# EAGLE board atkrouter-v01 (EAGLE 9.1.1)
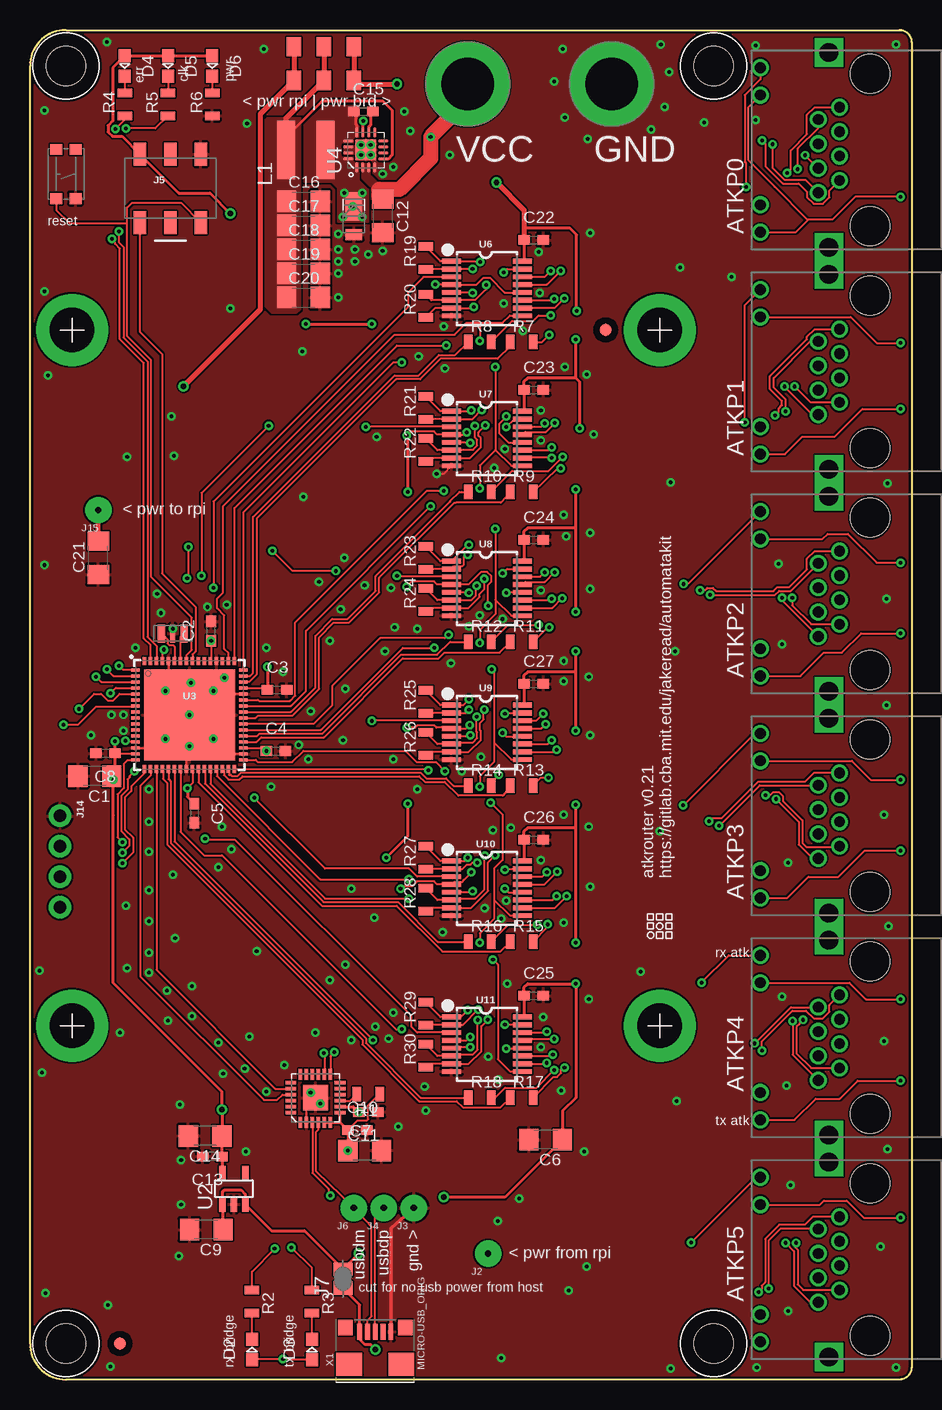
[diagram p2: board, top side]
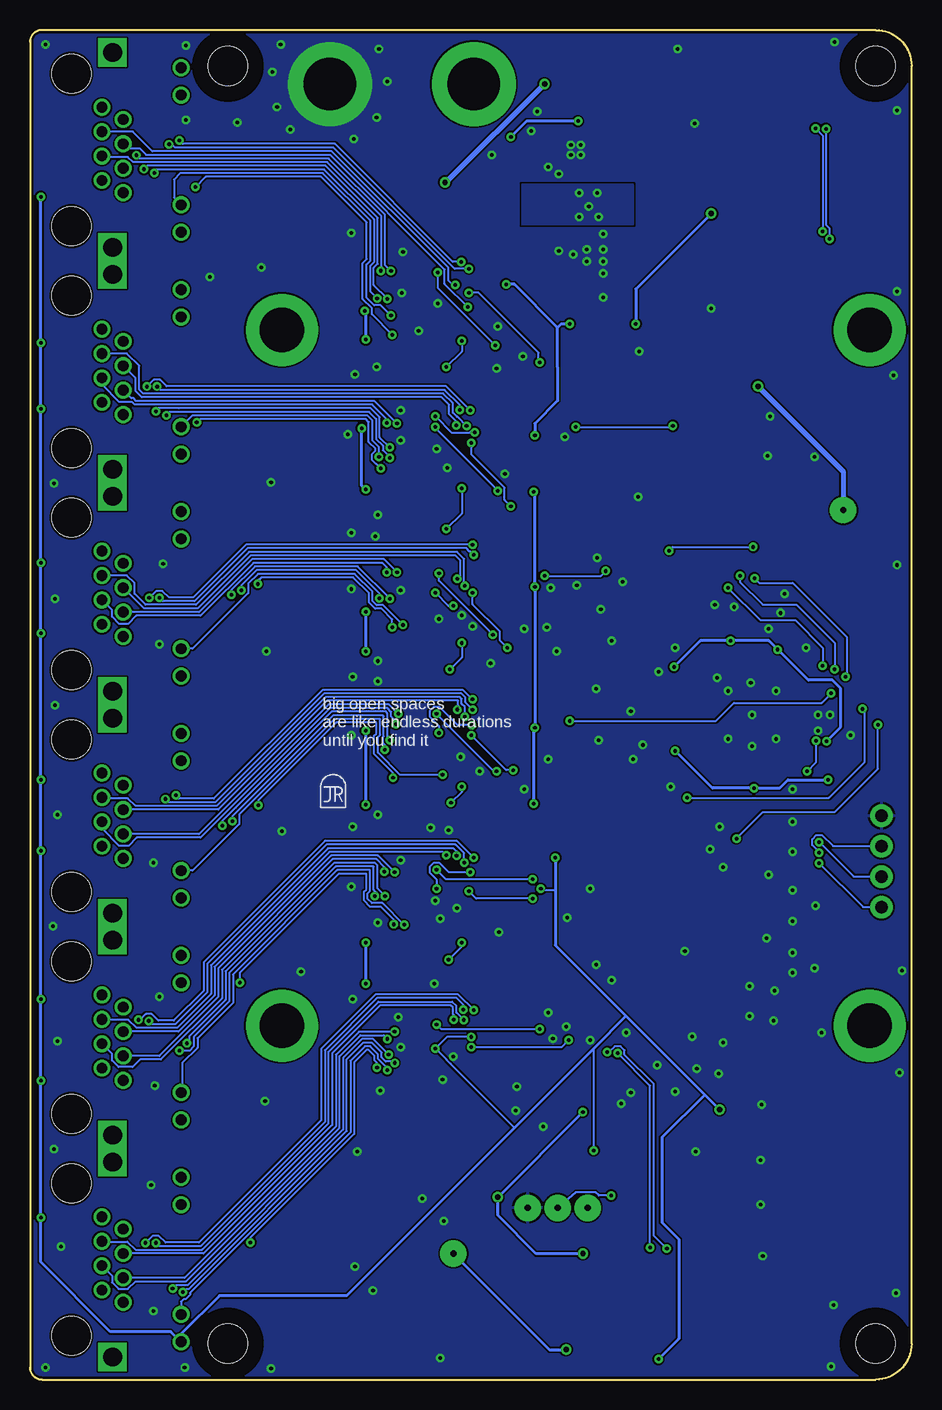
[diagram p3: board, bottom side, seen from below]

Size 73.5 x 112.5 mm. Coordinates in mm from the lower left corner, seen from the top.
Outline: 72.5,0 3,0 arc-90 0,3 0,109.5 arc-90 3,112.5 72.5,112.5 arc-90 73.5,111.5 73.5,1 arc-90 72.5,0
Copper layers (1*16): Top 0.035mm / dielectric 1.5mm / Bottom 0.035mm
Design rules "default *": minimum track width 6mil, minimum drill 0.3mm, track to track 6mil, track to pad 6mil, pad to pad 6mil, via to via 6mil, smd to smd 6mil, copper to edge 8mil, drill to drill 6mil, minimum pad ring 10mil, minimum via ring 8mil, stop-mask expansion 4mil, vias tented up to drill 25mil, thermal gap 8mil

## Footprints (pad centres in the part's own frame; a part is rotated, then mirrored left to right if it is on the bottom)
1206 = smd 1.6 x 1.8: 1 -1.4,0; 2 1.4,0
0603-CAP = smd 0.96 x 0.8: 1 -0.8,0; 2 0.8,0
SOD-123HE = smd 2.4 x 1.4: P$1 0.8,0 | smd 0.9 x 1.4: P$2 -1.55,0
LED0805 = smd 1.1 x 1: 1 -0.85,0; 2 0.85,0
FIDUCIAL_1MM = smd 1 x 1: 1 0,0
POGO = drill 0.51 pad 2.184: P$1 0,0
PDI_2X3_SMD = smd 1.02 x 1.9: 1 -2.54,-2.85; 2 -2.54,2.85; 3 0,-2.85; 4 0,2.85; 5 2.54,-2.85; 6 2.54,2.85
SJFAB = smd 1.118 x 1.6: 1 -0.787,0; 2 0.787,0
PWRPAD_M3_STANDOFF = drill 4.4 pad 7: P$1 0,0
PWRPAD_M25_STANDOFF = drill 3.7 pad 6: P$1 0,0
1X04_NO_SILK = drill 1.016 pad 1.88: 1 0,0; 2 2.54,0; 3 5.08,0; 4 7.62,0
RJ45-LED-RJHSE-5381-UPTAB = drill 0.889: GRNN 6.858,6.604; GRNP 4.572,6.604; YLWN -4.572,6.604; YLWP -6.858,6.604 | drill 0.9: P$1 3.556,0; P$2 2.54,1.778; P$3 1.524,0; P$4 0.508,1.778; P$5 -0.508,0; P$6 -1.524,1.778; P$7 -2.54,0; P$8 -3.556,1.778 | drill 1.575 square: SHDL1 -8.128,0.889; SHDL2 8.128,0.889 | hole 3.251: -6.35,-2.54; 6.35,-2.54
NRS5020T4R7MMGJ = smd 4.9 x 1.5: 1 0,1.65; 2 0,-1.65
NPTH-3-25MM = hole 3.25: 0,0
0805 = smd 0.7 x 1.2: 1 -0.95,0; 2 0.95,0
TACT-SWITCH-KMR6 = smd 0.9 x 1: P$1 -2.05,0.8; P$2 2.05,0.8; P$3 -2.05,-0.8; P$4 2.05,-0.8
SLIDESWITCH-CL-SB-22A = smd 1.2 x 1.6: P$1 -2.5,1.4; P$2 0,1.4; P$3 2.5,1.4; P$4 -2.5,-1.4; P$5 0,-1.4; P$6 2.5,-1.4
SOT23-5 = smd 0.533 x 1.194: 1 -0.95,-1.306; 2 0,-1.306; 3 0.95,-1.306; 4 0.95,1.306; 5 -0.95,1.306
QFN-64-9X9MM = smd 0.7 x 0.275: 1 -4.5,3.75; 2 -4.5,3.25; 3 -4.5,2.75; 4 -4.5,2.25; 5 -4.5,1.75; 6 -4.5,1.25; 7 -4.5,0.75; 8 -4.5,0.25; 9 -4.5,-0.25; 10 -4.5,-0.75; 11 -4.5,-1.25; 12 -4.5,-1.75; 13 -4.5,-2.25; 14 -4.5,-2.75; 15 -4.5,-3.25; 16 -4.5,-3.75; 33 4.5,-3.75; 34 4.5,-3.25; 35 4.5,-2.75; 36 4.5,-2.25; 37 4.5,-1.75; 38 4.5,-1.25; 39 4.5,-0.75; 40 4.5,-0.25; 41 4.5,0.25; 42 4.5,0.75; 43 4.5,1.25; 44 4.5,1.75; 45 4.5,2.25; 46 4.5,2.75; 47 4.5,3.25; 48 4.5,3.75 | smd 0.275 x 0.7: 17 -3.75,-4.5; 18 -3.25,-4.5; 19 -2.75,-4.5; 20 -2.25,-4.5; 21 -1.75,-4.5; 22 -1.25,-4.5; 23 -0.75,-4.5; 24 -0.25,-4.5; 25 0.25,-4.5; 26 0.75,-4.5; 27 1.25,-4.5; 28 1.75,-4.5; 29 2.25,-4.5; 30 2.75,-4.5; 31 3.25,-4.5; 32 3.75,-4.5; 49 3.75,4.5; 50 3.25,4.5; 51 2.75,4.5; 52 2.25,4.5; 53 1.75,4.5; 54 1.25,4.5; 55 0.75,4.5; 56 0.25,4.5; 57 -0.25,4.5; 58 -0.75,4.5; 59 -1.25,4.5; 60 -1.75,4.5; 61 -2.25,4.5; 62 -2.75,4.5; 63 -3.25,4.5; 64 -3.75,4.5 | smd 7.6 x 7.6: P$1 0,0
QFN16-3X3-TI-RTE = smd 0.85 x 0.3: 1 -1.475,0.75; 2 -1.475,0.25; 3 -1.475,-0.25; 4 -1.475,-0.75; 9 1.475,-0.75; 10 1.475,-0.25; 11 1.475,0.25; 12 1.475,0.75 | smd 0.3 x 0.85: 5 -0.75,-1.475; 6 -0.25,-1.475; 7 0.25,-1.475; 8 0.75,-1.475; 13 0.75,1.475; 14 0.25,1.475; 15 -0.25,1.475; 16 -0.75,1.475 | smd 1.7 x 1.7: TH 0,0
QFN-24_ALT2 = smd 0.9 x 0.3: 1 -2.05,1.25; 2 -2.05,0.75; 3 -2.05,0.25; 4 -2.05,-0.25; 5 -2.05,-0.75; 6 -2.05,-1.25; 13 1.95,-1.25; 14 1.95,-0.75; 15 1.95,-0.25; 16 1.95,0.25; 17 1.95,0.75; 18 1.95,1.25 | smd 0.3 x 0.9: 7 -1.25,-2.05; 8 -0.75,-2.05; 9 -0.25,-2.05; 10 0.25,-2.05; 11 0.75,-2.05; 12 1.25,-2.05; 19 1.25,2.05; 20 0.75,2.05; 21 0.25,2.05; 22 -0.25,2.05; 23 -0.75,2.05; 24 -1.25,2.05 | smd 2.1 x 2.1: EP 0,0
TSSOP16 = smd 0.4 x 1.6: 1 -2.225,-2.85; 2 -1.575,-2.85; 3 -0.925,-2.85; 4 -0.275,-2.85; 5 0.375,-2.85; 6 1.025,-2.85; 7 1.675,-2.85; 8 2.325,-2.85; 9 2.325,3.05; 10 1.675,3.05; 11 1.025,3.05; 12 0.375,3.05; 13 -0.275,3.05; 14 -0.925,3.05; 15 -1.575,3.05; 16 -2.225,3.05
DX4R005HJ5 = smd 0.4 x 1.35: D+ 0,1.6; D- -0.65,1.6; GND 1.3,1.6; ID 0.65,1.6; VBUS -1.3,1.6 | smd 1.2 x 1.3: GND@1 -2.5,1.95; GND@2 2.5,1.95 | smd 2.15 x 1.9: GND@3 -2.175,-1.1; GND@4 2.175,-1.1
RES_PRQC = smd 0.6 x 1.5: 1 -0.95,0; 3 0.95,0 | smd 0.4 x 1.5: 2 0,0

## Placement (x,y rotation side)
C1  10uF  [1206]  5.4,50.3 180 top
C2  0.1uF  [0603-CAP]  15.1,62.4 90 top
C3  0.1uF  [0603-CAP]  20.6,57.5 0 top
C4  0.1uF  [0603-CAP]  20.5,52.4 0 top
C5  0.1uF  [0603-CAP]  13.7,47.2 270 top
C6  10uF  [1206]  43,20 180 top
C7  10uF  [1206]  27.9,19.1 0 top
C8  0.1uF  [0603-CAP]  6.3,52.2 180 top
C9  10uF  [1206]  14.7,12.5 180 top
C10  0.1uF  [0603-CAP]  27.3,20.8 0 top
C11  0.1uF  [0603-CAP]  28.2,22.3 180 top
C12  10uF  [1206]  29.4,97 270 top
C13  0.1uF  [0603-CAP]  15.2,18.6 180 top
C14  10uF  [1206]  14.6,20.3 180 top
C15  0.1uF  [0603-CAP]  27.8,105.7 0 top
C16  10uF  [1206]  22.8,98.2 0 top
C17  10uF  [1206]  22.8,96.2 0 top
C18  10uF  [1206]  22.8,94.2 0 top
C19  10uF  [1206]  22.8,92.2 0 top
C20  10uF  [1206]  22.8,90.2 0 top
C21  10uF  [1206]  5.7,68.5 90 top
C22  0.1uF  [0603-CAP]  42,95 0 top
C23  0.1uF  [0603-CAP]  42,82.5 0 top
C24  0.1uF  [0603-CAP]  42,70 0 top
C25  0.1uF  [0603-CAP]  42,32 0 top
C26  0.1uF  [0603-CAP]  42,45 0 top
C27  0.1uF  [0603-CAP]  42,58 0 top
D1  [SOD-123HE]  27,97 90 top
D2  LED0805RX  [LED0805]  18.5,2.5 90 top
D3  LED0805TX  [LED0805]  23.5,2.5 90 top
D4  LED0805RX  [LED0805]  7.9,109.5 270 top
D5  LED0805RX  [LED0805]  11.5,109.5 270 top
D6  LED0805RX  [LED0805]  15.2,109.5 270 top
J1  FIDUCIAL  [FIDUCIAL_1MM]  7.5,3 0 top
J2  POGO  [POGO]  38.2,10.5 0 top
J3  POGO  [POGO]  32,14.3 0 top
J4  POGO  [POGO]  29.5,14.3 0 top
J5  [PDI_2X3_SMD]  11.7,99.3 0 top
J6  POGO  [POGO]  27,14.3 0 top
J7  SOLDER_JUMPER  [SJFAB]  26.1,8.4 90 top
J8  PWRPADM3-STANDOFF  [PWRPAD_M3_STANDOFF]  36.5,108 0 top
J9  PWRPADM3-STANDOFF  [PWRPAD_M3_STANDOFF]  48.5,108 0 top
J10  PWRPADM2.5_STANDOFF  [PWRPAD_M25_STANDOFF]  52.5,29.5 0 top
J11  PWRPADM2.5_STANDOFF  [PWRPAD_M25_STANDOFF]  52.5,87.5 0 top
J12  PWRPADM2.5_STANDOFF  [PWRPAD_M25_STANDOFF]  3.5,87.5 0 top
J13  PWRPADM2.5_STANDOFF  [PWRPAD_M25_STANDOFF]  3.5,29.5 0 top
J14  [1X04_NO_SILK]  2.5,47 270 top
J15  POGO  [POGO]  5.7,72.48 0 top
J16  ATK-RS48PHYVERJ45LEDTABUP  [RJ45-LED-RJHSE-5381-UPTAB]  67.5,102.5 90 top
J17  ATK-RS48PHYVERJ45LEDTABUP  [RJ45-LED-RJHSE-5381-UPTAB]  67.5,84 90 top
J18  ATK-RS48PHYVERJ45LEDTABUP  [RJ45-LED-RJHSE-5381-UPTAB]  67.5,65.5 90 top
J19  ATK-RS48PHYVERJ45LEDTABUP  [RJ45-LED-RJHSE-5381-UPTAB]  67.5,47 90 top
J20  ATK-RS48PHYVERJ45LEDTABUP  [RJ45-LED-RJHSE-5381-UPTAB]  67.5,28.5 90 top
J21  ATK-RS48PHYVERJ45LEDTABUP  [RJ45-LED-RJHSE-5381-UPTAB]  67.5,10 90 top
J22  FIDUCIAL  [FIDUCIAL_1MM]  48,87.5 0 top
L1  4.7uH  [NRS5020T4R7MMGJ]  23,102.5 90 top
M1  M3-NPTH  [NPTH-3-25MM]  57,109.5 0 top
M2  M3-NPTH  [NPTH-3-25MM]  57,3 0 top
M3  M3-NPTH  [NPTH-3-25MM]  3,109.5 0 top
M4  M3-NPTH  [NPTH-3-25MM]  3,3 0 top
MP1  JRTOMBSTONE  [JRTOMBSTONE]  48.17,48.68 0 bottom
R1  10k  [0805]  28.2,23.8 180 top
R2  1k  [0805]  18.5,6.5 270 top
R3  1k  [0805]  23.5,6.5 270 top
R4  470R  [0805]  7.9,106.3 90 top
R5  470R  [0805]  11.5,106.3 90 top
R6  470R  [0805]  15.2,106.3 90 top
R7  470R  [0805]  41,86.5 0 top
R8  470R  [0805]  37.5,86.5 0 top
R9  470R  [0805]  41,74 0 top
R10  470R  [0805]  37.5,74 0 top
R11  470R  [0805]  41,61.5 0 top
R12  470R  [0805]  37.5,61.5 0 top
R13  470R  [0805]  41,49.5 0 top
R14  470R  [0805]  37.5,49.5 0 top
R15  470R  [0805]  41,36.5 0 top
R16  470R  [0805]  37.5,36.5 0 top
R17  470R  [0805]  41,23.5 0 top
R18  470R  [0805]  37.5,23.5 0 top
R19  120R  [0805]  33,93.5 90 top
R20  120R  [0805]  33,89.5 90 top
R21  120R  [0805]  33,81 90 top
R22  120R  [0805]  33,77.5 90 top
R23  120R  [0805]  33,68.5 90 top
R24  120R  [0805]  33,65 90 top
R25  120R  [0805]  33,56.5 90 top
R26  120R  [0805]  33,53 90 top
R27  120R  [0805]  33,43.5 90 top
R28  120R  [0805]  33,40 90 top
R29  120R  [0805]  33,30.5 90 top
R30  120R  [0805]  33,27 90 top
S1  2-8X4-5_SWITCH  [TACT-SWITCH-KMR6]  3,100.5 270 top
S2  SLIDE-SWITCHSMT  [SLIDESWITCH-CL-SB-22A]  24.5,109.7 0 top
U1  RASPBERRYPI-3BPLUS  [RASPBERRYPI-3BPLUS]  0,6 0 top
U2  VREG-AP2112  [SOT23-5]  17,15.9 0 top
U3  ATXMEGA_A3UQFN  [QFN-64-9X9MM]  13.3,55.4 0 top
U4  BUCK-TS30011-12-13QFN  [QFN16-3X3-TI-RTE]  28,102.5 90 top
U5  CP2102N  [QFN-24_ALT2]  23.8,23.5 90 top
U6  RS485-2BY2-SN75C1168PWR  [TSSOP16]  38,91 270 top
U7  RS485-2BY2-SN75C1168PWR  [TSSOP16]  38,78.5 270 top
U8  RS485-2BY2-SN75C1168PWR  [TSSOP16]  38,66 270 top
U9  RS485-2BY2-SN75C1168PWR  [TSSOP16]  38,54 270 top
U10  RS485-2BY2-SN75C1168PWR  [TSSOP16]  38,41 270 top
U11  RS485-2BY2-SN75C1168PWR  [TSSOP16]  38,28 270 top
U$2  CBA-LOGO  [CBA-SILK-LOGO]  52.5,37.8 90 top
X1  MICRO-USB_ORIG  [DX4R005HJ5]  28.79,2.38 0 top
Y1  RESONATORPQRC  [RES_PRQC]  11.9,62.2 180 top

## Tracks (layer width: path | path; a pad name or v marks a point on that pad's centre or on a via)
5VBUCK
  Top 0.254: L1.1 21.35,103.55 24.4,106.6 29.4,106.6 30.18,105.82 30.18,102.05 29.88,101.75 U4.5
  Top 0.406: S2.P$2 S2.P$5 21.35,105.15 L1.1
  pour Top (no thermals): 22.5,105.2 22.5,89.2 22.2,88.9 20.2,88.9 19.6,89.5 19.6,105 19.8,105.2
+3V3  (via drill 0.3, 0.45)
  Top 0.152: U6.12 39.58,90.62 38.36,91.84 37.8,91.84 37.23,91.28 U6.4 33.83,91.28 v33.8,91.31 | v36.42,78.96 36.24,78.78 U7.4 33.95,78.78 33.7,79.03 31.73,79.03 v31.4,78.7 | v39.7,80.3 39.7,80.22 39.12,79.64 39.12,78.88 39.9,78.1 41.02,78.1 U7.12 | U8.12 39.73,65.62 v39.7,65.6 | v38.2,64.5 38.2,66.24 38.46,66.51 38.46,66.99 38.12,67.33 37.61,67.33 36.55,66.28 U8.4 33.95,66.28 33.7,66.53 31.83,66.53 v31.4,66.1 | v36.66,54.56 36.37,54.27 U9.4 35.08,54.34 33.88,54.34 33.7,54.53 32.3,54.53 32.12,54.34 v31.4,54.34 | v39.4,53.9 39.67,53.62 U9.12 | v36.8,42.28 36.18,41.66 36.18,41.63 36.05,41.5 35.37,41.5 U10.4 33.95,41.27 33.7,41.53 32.25,41.53 31.84,41.12 31.12,41.12 v30.9,40.9 | v39.6,40.9 39.88,40.62 U10.12 | U11.4 36.42,28.27 v36.7,28.56 | v39.7,27.6 41.02,27.6 U11.12 | C10.1 27.3,21.6 28.1,21.6 28.2,21.7 28.2,22.85 R1.1 | D2.1 18.55,1.7 v21.1,1.7 23.45,1.7 D3.1 | U3.61 11.05,60.75 v11.15,60.85 | C2.1 15.1,59.95 U3.53 | U3.45 19.65,57.65 C3.1 | C8.1 8.75,52.2 U3.15 | U3.35 19.45,52.65 C4.1 | U3.25 13.55,49.72 v13.13,49.3 | J16.GRNP 59.9,106.08 59.9,101.63 62.1,99.43 64.83,96.7 64.9,96.7 | v72.6,98.6 68.8,98.6 66.9,96.7 64.9,96.7 | 64.9,96.7 63.84,95.64 J16.YLWP | J17.GRNP 68.43,88.57 70.6,86.4 v72.6,86.4 | J17.YLWP 62.94,77.14 64.4,78.6 67.1,78.6 69.4,80.9 v72.6,80.9 | J18.GRNP 66.07,70.07 66.5,70.5 68.2,70.5 70.6,68.1 v72.6,68.1 | J18.YLWP 64.24,58.64 66.2,60.6 67.7,60.6 69.3,62.2 v72.6,62.2 | J19.GRNP 68.53,51.57 70.1,50 v72.6,50 | J19.YLWP 63.14,40.14 64.9,41.9 67.4,41.9 69.6,44.1 v72.6,44.1 | J20.GRNP 68.33,33.07 69.7,31.7 v72.6,31.7 | J20.YLWP 63.74,21.64 65.5,23.4 67.5,23.4 69,24.9 v72.6,24.9
  Top 0.152: J21.GRNP 65.87,14.57 66.2,14.9 68.1,14.9 69.5,13.5 v72.6,13.5
  Top 0.254: U5.5 U5.6 25.75,21.45 | U5.7 25.85,21.55 25.75,21.45 | 25.75,21.45 25.85,21.45 C10.1 C7.1 | U2.5 16.05,18.55 C13.1 C14.1 v16,22.5 16,24 6.95,33.05 6.95,47.05 v6.95,50 6.95,50.45 C1.1 7.1,50.6 C8.1 v7.1,53.2 | D6.1 D5.1 D4.1 6.9,109.35 6.9,104.92 6.51,104.52 6.51,104 6.88,103.63 7.68,103.63 J5.2 12.41,98.9 15,98.9 v16.7,97.2 | v13.13,49.3 13.13,48.57 C5.1 | v19.8,59.4 C3.1 | v29.7,43.5 31.5,45.3 v31.5,48 | v31.5,74 31.5,78.6 v31.4,78.7 | v23,88 v28.5,88
  Bottom 0.152: v36.42,78.96 36.81,78.96 36.86,78.91 38.31,78.91 v39.7,80.3 | v39.7,65.6 38.6,64.5 v38.2,64.5 | v36.66,54.56 37.84,54.56 39.36,56.08 39.84,56.08 40.18,55.74 40.18,55.26 39.4,54.48 v39.4,53.9 | v39.6,40.9 39.6,41.68 40.18,42.26 40.18,42.74 39.84,43.08 39.36,43.08 38.56,42.28 v36.8,42.28 | v36.7,28.56 38.74,28.56 v39.7,27.6 38.78,26.68 38.78,26.66 38.44,26.32 38.42,26.32 33.1,21 | C7.1 26.5,27.6 | v30.9,40.9 30.8,40.8 29.7,40.8
  Bottom 0.254: v31.4,78.7 31.4,79.7 29.51,81.59 29.51,84.3 29.51,84.39 29.51,87.71 | v29.7,43.5 29.7,40.8 29.7,36.2 23.8,30.3 | 23.8,30.3 17.25,23.75 | 17.25,23.75 v16,22.5 | 23.8,30.3 26.5,27.6 33.1,21 47.1,7 57.7,7 60.9,3.8 J21.YLWP 61.75,4 66.8,4 72.6,9.8 v72.6,13.5 v72.6,24.9 v72.6,31.7 v72.6,44.1 v72.6,50 v72.6,62.2 v72.6,68.1 v72.6,80.9 v72.6,86.4 v72.6,98.6 | 17.25,23.75 20.8,20.2 20.8,13.1 19.4,11.7 19.4,3.4 v21.1,1.7 | C4.1 16.6,49.3 v13.13,49.3 11,49.3 10.3,50 v6.95,50 | v7.1,53.2 5.9,54.4 5.9,57.6 6.6,58.3 8.6,58.3 v11.15,60.85 11.9,61.6 C2.1 17.6,61.6 v19.8,59.4 | v33.8,91.31 33.11,91.31 29.51,87.71 | v31.5,48 31.5,54.24 v31.4,54.34 v31.4,66.1 31.4,73.9 v31.5,74 | v16.7,97.2 23,90.9 v23,88 | v28.5,88 29.21,88 29.51,87.71
  other vias: 26.5,19.1 19.7,52.4 15.1,61.6
+5V  (via drill 0.3, 0.45)
  Top 0.254: C9.1 16.05,12.75 U2.1 16.05,15.65 16.2,15.8 17.6,15.8 17.95,15.45 U2.3 20.14,12.4 22.89,12.4 J7.2 | U6.16 41.2,93.38 C22.1 41.2,95.7 | U11.16 41.2,30.38 C25.1 41.2,32.7 41.5,33 v45.5,33 45.5,23.5 44.4,22.4 C6.1 39.6,15.2 v34.5,15.2 | U10.16 41.2,43.38 C26.1 41.2,45.7 41.5,46 45.5,46 | U9.16 41.2,56.38 C27.1 41.2,58.7 41.5,59 45.5,59 | U8.16 41.2,68.38 C24.1 41.2,70.7 41.5,71 45.5,71 | U7.16 41.2,80.88 C23.1 41.2,83.2 41.5,83.5 45.5,83.5 | U5.8 26.95,22.75 C11.2 | J7.2 27.4,10.49 v27.4,10.5 | J7.2 J7.1 27.49,6.22 X1.VBUS 27.49,3.36 27.95,2.9 28.4,2.9 v28.8,2.5 | 41.2,96 45,96 45.58,95.42 v45.58,89.08 | v45.5,36.4 45.5,46 | 45.5,46 v45.5,47.9 | v45.5,54.1 45.5,59 | 45.5,59 v45.5,60.7 | v45.5,64 45.5,71 | 45.5,71 v45.5,74.2 | v45.84,79.3 45.84,83.16 45.5,83.5 | 45.5,83.5 v45.5,86.7
  Top 0.406: S2.P$3 S2.P$6 27.3,108 v30.6,108 | v38.9,99.8 41.2,97.5 41.2,96 C22.1
  Bottom 0.254: C11.2 v34.5,15.2 34.5,13.7 31.3,10.5 v27.4,10.5 | J2.P$1 30.2,2.5 v28.8,2.5 | v45.5,33 v45.5,36.4 | v45.5,47.9 v45.5,54.1 | v45.5,60.7 v45.5,64 | v45.5,74.2 45.84,74.54 v45.84,79.3 | v45.5,86.7 45.5,89 v45.58,89.08
  Bottom 0.406: v30.6,108 38.8,99.8 v38.9,99.8
  other vias: 27.4,22.3
ATK0-CLKIN  (via drill 0.3)
  Top 0.152: U6.3 35.12,91.9 32.8,91.9 31.5,90.6 31.5,89.4 15.3,73.2 v15.3,66 | U3.1 7.75,59.15 v7.4,59.5
  Bottom 0.152: v15.3,66 12.6,63.3 9.7,63.3 7.4,61 v7.4,59.5
ATK0-RX  (via drill 0.3)
  Top 0.152: U3.48 17.8,72.3 30.3,84.8 v31,84.8 | v36.9,90.6 35.17,90.6 U6.5
  Bottom 0.152: v31,84.8 31.1,84.9 31.1,85.6 36.1,90.6 v36.9,90.6
ATK0-RXLED
  Top 0.152: R7.1 40.05,86.15 38.99,85.09 34.23,85.09 32.53,83.39 30.53,83.39 18.91,71.77 18.91,58.77 18.28,58.15 U3.46
ATK0-TX  (via drill 0.3)
  Top 0.152: U3.49 17.05,72.65 30.6,86.2 v34.7,86.2 | v39.5,92.3 39.77,92.58 U6.15
  Bottom 0.152: v34.7,86.2 39.5,91 v39.5,92.3
ATK0-TXLED
  Top 0.152: U3.47 18.35,58.65 18.6,58.9 18.6,71.9 30.4,83.7 32.4,83.7 34.1,85.4 35.45,85.4 R8.1
ATK1-CLKIN  (via drill 0.3)
  Top 0.152: U7.3 28.02,79.42 v28,79.4 | v6.4,59.2 6.95,58.65 U3.2 | v19.9,79.5 14.3,73.9 v14.3,67
  Bottom 0.152: v28,79.4 20,79.4 v19.9,79.5 | v6.4,59.2 6.4,61.4 9.6,64.6 12.4,64.6 14.3,66.5 v14.3,67
ATK1-RX  (via drill 0.3)
  Top 0.152: U3.42 21.75,56.15 23,57.4 23,62.4 v33.4,72.8 | v36.7,78.1 35.17,78.1 U7.5
  Bottom 0.152: v33.4,72.8 33.92,73.32 33.92,74.34 36.7,77.12 v36.7,78.1
ATK1-RXLED
  Top 0.152: R9.1 39.25,73.1 35.5,73.1 35.38,73.1 29.12,66.84 29.12,65.62 26.6,63.1 25.33,63.1 24.11,61.87 24.11,57.57 21.88,55.34 19,55.34 18.8,55.15 U3.40
ATK1-TX  (via drill 0.3)
  Top 0.152: U3.43 19.02,56.65 19.1,56.57 21.67,56.57 22.11,57.01 22.11,63.11 33.1,74.1 v34.5,74.1 | v39.7,79.4 40.38,80.08 U7.15
  Bottom 0.152: v34.5,74.1 39.7,79.3 v39.7,79.4
ATK1-TXLED
  Top 0.152: U3.41 21.75,55.65 23.8,57.7 23.8,62 25.2,63.41 26.47,63.41 28.81,65.74 28.81,66.97 35.03,73.18 35.03,73.23 35.8,74 36,74 R10.1
ATK2-CLKIN  (via drill 0.3)
  Top 0.152: U8.3 30.68,66.92 v30.6,67 | v25.5,67.4 21.9,67.4 v20.2,69.1 | v13.2,69.4 13.2,67 v13.1,66.8 | v5.5,58.6 5.95,58.15 U3.3
  Bottom 0.152: v30.6,67 25.9,67 v25.5,67.4 | v20.2,69.1 19.9,69.4 v13.2,69.4 | v13.1,66.8 12.7,66.4 9.9,66.4 5.4,61.9 5.4,58.7 v5.5,58.6
ATK2-RX  (via drill 0.3)
  Top 0.152: U3.38 24.25,54.15 31.1,61 v33.7,61 | v36.6,65.6 35.17,65.6 U8.5
  Bottom 0.152: v33.7,61 34.32,61.62 34.32,62.34 36.6,64.62 v36.6,65.6
ATK2-RXLED
  Top 0.152: U3.36 18.88,53.15 19.27,53.54 24.5,53.54 31.08,60.11 34.07,60.11 34.55,60.6 39.15,60.6 R11.1
ATK2-TX  (via drill 0.3)
  Top 0.152: v34.9,62.1 34.6,61.8 29.2,61.8 25.2,57.8 25.2,56.2 23.65,54.65 U3.39 | v39.4,67.2 39.77,67.58 U8.15
  Bottom 0.152: v34.9,62.1 39.4,66.6 v39.4,67.2
ATK2-TXLED
  Top 0.152: U3.37 18.95,53.65 19.14,53.84 24.38,53.84 30.95,60.42 33.94,60.42 35.02,61.5 R12.1
ATK3-CLKIN  (via drill 0.3)
  Top 0.152: U9.3 28.52,54.92 v28.5,54.9 | v6.7,57.2 7.15,57.65 U3.4
  Bottom 0.152: v28.5,54.9 16.3,54.9 14.8,56.4 7.5,56.4 v6.7,57.2
ATK3-RX  (via drill 0.3)
  Top 0.152: U3.32 33.1,50.9 v33.2,50.8 | v36.7,53.7 36.62,53.62 U9.5
  Bottom 0.152: v33.2,50.8 33.8,50.8 v36.7,53.7
ATK3-RXLED
  Top 0.152: U3.30 16.18,50.77 16.18,50.38 16.55,50.02 17.45,50.02 17.72,50.29 32.46,50.29 32.93,49.81 34.57,49.81 35.72,48.67 39.42,48.67 R13.1
ATK3-TX  (via drill 0.3)
  Top 0.152: U3.33 18.82,51.65 19,51.47 21.87,51.47 22.8,52.4 31.3,52.4 32.23,51.47 33.83,51.47 v34.6,50.7 | v39.6,55.5 39.67,55.58 U9.15
  Bottom 0.152: v34.6,50.7 34.8,50.7 v39.6,55.5
ATK3-TXLED
  Top 0.152: U3.31 16.6,50.85 16.6,50.4 16.74,50.4 16.82,50.32 17.32,50.32 17.59,50.59 32.58,50.59 33.06,50.12 34.7,50.12 35.32,49.5 R14.1
ATK4-CLKIN  (via drill 0.3)
  Top 0.152: U10.3 32.27,41.92 31.6,42.6 24.6,42.6 v18.7,48.5 | v4.1,55.9 5.35,57.15 5.93,57.15 6.46,56.62 6.94,56.62 7.47,57.15 U3.5
  Bottom 0.152: v18.7,48.5 6.9,48.5 3.9,51.5 3.9,55.7 v4.1,55.9
ATK4-RX  (via drill 0.3)
  Top 0.152: U3.28 15.05,49.65 24.6,40.1 v31.6,40.1 | v36.9,40.7 36.83,40.62 U10.5
  Bottom 0.152: v31.6,40.1 36.3,40.1 v36.9,40.7
ATK4-RXLED
  Top 0.152: U3.26 14.05,49.79 24.35,39.49 30.57,39.49 34.39,35.67 39.22,35.67 R15.1
ATK4-TX  (via drill 0.3)
  Top 0.152: U3.29 15.6,50.85 15.6,50.3 24.2,41.7 v31.6,41.7 | v39.6,42.5 39.67,42.58 U10.15
  Bottom 0.152: v31.6,41.7 38.8,41.7 v39.6,42.5
ATK4-TXLED
  Top 0.152: U3.27 14.6,50.85 14.6,49.67 24.47,39.8 30.7,39.8 33.99,36.5 R16.1
ATK5-CLKIN  (via drill 0.3)
  Top 0.152: v14.6,45.1 14.6,45 17.1,45 31.8,30.3 31.8,29.4 32.27,28.93 U11.3 | v2.8,54.6 4,54.6 5.5,56.1 8.75,56.1 U3.7
  Bottom 0.152: v14.6,45.1 12.4,47.3 6.4,47.3 2.8,50.9 v2.8,54.6
ATK5-RX  (via drill 0.3)
  Top 0.152: U3.22 12.05,44.85 v28.6,28.3 | v36.7,27.7 35.23,27.7 U11.5
  Bottom 0.152: v28.6,28.3 29.2,27.7 v36.7,27.7
ATK5-RXLED
  Top 0.152: U3.20 11.1,50.85 11.1,50.07 11.44,49.73 11.44,44.6 27.71,28.32 27.71,27.93 32.45,23.2 35.58,23.2 36.1,22.67 39.22,22.67 R17.1
ATK5-TX  (via drill 0.3)
  Top 0.152: U3.23 12.55,45.65 14.5,43.7 16,43.7 30.5,29.2 v31,29.2 | v39.6,29.6 41.02,29.6 U11.15
  Bottom 0.152: v39.6,29.6 39.2,29.2 v31,29.2
ATK5-TXLED
  Top 0.152: U3.21 11.55,50.05 11.74,49.85 11.74,44.72 28.02,28.45 28.02,28.06 32.58,23.5 R18.1
ATK-CLKOUT  (via drill 0.3)
  Top 0.152: 37.6,88.1 36.4,88.1 35.4,87.1 30.4,87.1 16.1,72.8 16.1,65.6 15.6,65.1 15.6,64.3 16.2,63.7 16.2,60.9 16.55,60.55 U3.50 | 37.6,88.1 39.4,88.1 40,88.7 41.02,88.7 U6.9 | 37.6,88.1 37.5,88 v37.5,86.6 | v38.8,84.4 38.8,77.5 | U7.9 40.12,76.17 38.8,77.5 | 38.8,77.5 37.5,76.2 v37.5,74.3 | v38.8,70.9 38.8,65 | U8.9 40.12,63.67 38.8,65 | 38.8,65 38.8,63.8 37.5,62.5 v37.5,61.4 | v38.5,59.2 38.7,59 38.7,53.1 | U9.9 40.12,51.67 38.7,53.1 | 38.7,53.1 38.7,51.5 37.5,50.3 v37.5,49.4 | v38.4,48.09 39.4,47.09 39.4,43.3 38.7,42.6 38.7,40 | U10.9 40.02,38.67 38.7,40 | 38.7,40 38.7,38.4 37.5,37.2 v37.5,36.4 | v38.6,35 39,34.6 39,26.7 40.02,25.68 U11.9
  Bottom 0.152: v37.5,86.6 37.5,85.7 v38.8,84.4 | v37.5,74.3 37.5,72.2 v38.8,70.9 | v37.5,61.4 37.5,60.2 v38.5,59.2 | v37.5,49.4 37.5,48.99 v38.4,48.09 | v37.5,36.4 37.5,36.1 v38.6,35
BUCKBST
  Top 0.254: U4.10 28.25,104.45 28.43,104.64 28.43,105.53 C15.2
CLKRX-A  (via drill 0.3)
  Top 0.152: v36.9,92.6 35.17,92.6 U6.2 35.12,92.55 R19.1 | J16.P$8 64.65,100.01 62.9,100.01 61.9,101.01 v61.9,102.98
  Bottom 0.152: v36.9,92.6 38.1,92.6 48.2,102.7 61.4,102.7 61.68,102.98 v61.9,102.98
CLKRX-B  (via drill 0.3)
  Top 0.152: v37.53,93.18 37.49,93.22 U6.1 34.23,93.22 R19.2 | v61.04,103.28 61.32,103 61.32,101.16 62.77,99.71 64.1,99.71 64.79,99.02 64.79,98.56 65.34,98.01 66.11,98.01 66.66,98.56 66.66,99.11 J16.P$7
  Bottom 0.152: v37.53,93.18 38.25,93.18 48.07,103 60.76,103 v61.04,103.28
CLKRX-Y  (via drill 0.3)
  Top 0.152: v44.56,90.14 43.75,89.33 U6.10 | v63.14,100.59 63.42,100.87 63.42,102.45 64.79,103.83 64.79,105.43 65.42,106.06 J16.P$1
  Bottom 0.152: v44.56,90.14 45.15,90.72 45.15,92.8 44.81,93.13 44.81,96.71 48.97,100.87 63.1,100.87 63.14,100.83 v63.14,100.59
CLKTX-Z  (via drill 0.3)
  Top 0.152: U6.11 43.58,89.97 v43.7,90.1 | v64,100.9 64.03,100.93 64.03,102.64 65.72,104.33 J16.P$2
  Bottom 0.152: v43.7,90.1 44.84,91.24 44.84,92.68 44.51,93.01 44.51,96.84 48.85,101.18 63.72,101.18 v64,100.9
CPRX
  Top 0.152: U3.18 10.05,50.35 9.2,49.5 9.2,33.6 19.5,23.3 20.6,23.3 21.05,23.75 U5.21
CPRXLED  (via drill 0.3)
  Top 0.152: R2.1 18.5,9 v20.4,10.9 | v25.36,27.3 25.08,27.02 25.08,26.96 25.05,26.93 U5.13
  Bottom 0.152: v20.4,10.9 21.5,12 21.5,24.63 23.92,27.05 23.92,27.44 24.26,27.78 24.74,27.78 25.22,27.3 v25.36,27.3
CPTX
  Top 0.152: U3.19 10.55,34.15 20.45,24.25 U5.20
CPTXLED  (via drill 0.3)
  Top 0.152: R3.1 23.5,9.3 v21.8,11 | v24.5,27.2 24.55,27.15 U5.14
  Bottom 0.152: v21.8,11 21.8,24.5 v24.5,27.2
DBP1  (via drill 0.3)
  Top 0.152: U3.13 8.05,53.15 v7.96,53.24 | v8.7,50.7 8.3,50.3 8.3,50.2 8.13,50.03 8.13,49.18 7.61,48.66 7.61,45.71 8.28,45.04 8.28,44.48 v7.7,43.9
  Bottom 0.152: v7.96,53.24 7.96,51.44 v8.7,50.7 | v7.7,43.9 7.7,43.98 8.28,44.56 8.28,45.04 7.94,45.38 7.46,45.38 6.54,44.46 J14.2
DBP2  (via drill 0.3)
  Top 0.152: U3.16 8.75,51.6 8.1,51.6 7.83,51.33 7.83,49.3 7.31,48.78 7.31,45.19 v7.7,44.8
  Bottom 0.152: v7.7,44.8 4.82,41.92 J14.3
DBP3  (via drill 0.3)
  Top 0.152: U3.17 9.55,50.55 8.44,49.44 8.44,49.05 7.92,48.53 7.92,45.84 8.59,45.17 8.59,43.93 v7.7,43.04
  Bottom 0.152: v7.7,43.04 4.04,39.38 J14.4
DM
  Top 0.152: X1.D- 28.14,4.94 28.48,5.29 28.48,12.71 J6.P$1 23.86,17.34 23.86,20.66 24.05,20.85 U5.4
DP  (via drill 0.3)
  Top 0.152: X1.D+ 28.79,13.79 J4.P$1 | v25.04,15.34 24.88,15.49 24.88,15.88 23.55,17.22 U5.3
  Bottom 0.152: v25.04,15.34 26.07,15.34 26.35,15.62 27.98,15.62 J4.P$1
GND  (via drill 0.3)
  Top 0.152: U3.60 11.55,57.15 13.25,55.45 | 13.25,55.45 U3.P$1 | 12.3,54.4 v11.3,53.4 10.55,52.65 U3.14 | 12.3,54.4 13.25,55.35 | 13.25,55.35 U3.P$1 | 13.05,55.25 13.25,55.45 | 13.45,55.15 16.45,52.15 U3.34 | 13.45,55.15 13.25,55.35 | 13.45,55.15 15.45,57.15 15.5,57.15 15.55,57.2 | U5.2 23.05,23.55 v23.4,23.9 | U7.8 34.48,75.5 v33.9,75.5 | U3.P$1 v15.3,53.4 | U3.44 15.55,57.15 v15.3,57.4 | U3.24 13.05,52.85 13.1,52.9 13.1,53.6 12.3,54.4
  Top 0.305: X1.GND 30.09,12.59 J3.P$1
  other vias: 13.3,55.4 11.3,57.4 24.2,23 11.9,62.6 37.6,51.9 36,50.7 44.5,58.2 44.5,47.1 40.1,46 42.6,43.3 37.9,39.3 34.4,37.3 42.8,30.2 42.6,27.7 38.2,26.9 39.1,25 32.9,24.4 29.9,28.4 37.5,63.7 36.6,62.8 32.3,62.6 30.4,62.7 30.1,66 23.4,55.7 25,61.6 44.7,70.3 42.6,65.8 38.7,76 39.6,77.6 42.6,80.8 42.6,78.3 39.5,89.7 34.5,87.8 42.4,94 42.5,90.6 41.1,87.4 44.6,84.4 32.4,85.3 16.4,64.6 38.6,45.8 32.3,49.2 20.1,49.4 26.8,40.9 39.4,63.4 26.3,57.6 29.6,60.7 25.9,64.2 27.9,66.2 21.1,59 24.1,66.5 26.2,68.5 28.9,78.6 34.6,84.3 9.9,49.2 9.9,46.5 9.9,44 9.9,40.8 9.9,38.2 9.9,35.6 9.9,33.9 11.4,32.4 13.5,30.3 15.7,28.1 17.9,25.9 19.7,24 8,39.5 8.1,34.3 11.5,29.9 16.1,25.5 18.3,28.6 21.2,26.2 13.5,32.8 12.1,36.8 11.9,42.1 23.2,51.7 30.3,51.7 26.1,53.3 35.1,59.7 44.5,59.9 44.5,72.1 46.7,95.6 46.4,83.8 47,78.8 46.7,70.6 46.7,65.9 46.6,58.6 46.7,53.7 46.6,46.1 46.7,41.1 46.6,31.7 44.3,24.1 46.4,9.4 44.9,7.4 39,13.2 40.8,15.1 33,22.4 30.7,21.1 28.8,29.4 28.7,38.5 60.5,105 58.5,91.9 56.2,104.8 44.4,110.9 43.7,108.2 44.6,105.2 46.5,103.4 51.8,104.2 52.9,106.1 53.3,109 52.6,111.3 11.8,80.3 8.1,76.9 12,77 10.6,65.5 10.9,63.9 30.3,30.6 26.3,34.6 25,33.3 15.7,42.7 16.8,44.2 16,46.1 18.9,35.7 26.8,28.3 23.8,28.9 18,19 12.6,18.3 12.6,14.6 12.4,10.3 12.5,22.9 1.3,7.2 6.7,1.1 53.4,0.9 60.6,1 6.5,6.2 1,25.6 0.8,34.1 7.5,28.9 50.9,34 1.2,67.9 5.1,53.7 7.8,55.4 8.8,61 14.8,64.4 19.7,61 13.4,58.1 13.3,52.8 16.2,58.5 6.8,55.4 7.8,54.1 22.4,52.9 1.5,83.7 1.2,90.7 1.2,105.8 6.4,111.5 60.5,111.2 54.2,92.7 53.4,74.8 16.7,89.3 22.7,85.7 22.8,73.6 53.8,60.7 52.5,45.7 39.3,1.8 27.6,102.9 28.4,102.9 28.4,102.1 27.6,102.1 29.4,100.5 30.3,101.1 31.7,104.1 31.2,105.7 35,102.1 25.7,95.5 25.7,94.2 27.1,94.2 28.2,93.8 29.4,94.1 25.7,93.2 25.7,92.2 25.7,90.2 27.1,93.2 72.2,111.3 44.5,38.1 39.3,38.4 39.7,39.9 39.8,33 62.7,61.3 62.4,68 71.5,74.7 71.4,65.1 71.4,56.2 63.2,43.1 71.2,47.1 71.6,37.8 62.7,31.9 63.1,24.5 71.2,28.2 71.5,19.2 63.4,16.2 63.2,5.7 70.9,11.1 72.2,1 53.9,23.2 46.2,19 18.1,104.7 19.5,110.9
  pour Bottom (rank 6): -6,122 84,122 84,-1.5 -6,-1.5
  pour Top (rank 6): -4.5,120.5 83,120.5 83,-0.5 -4.5,-0.5
  pour Top (rank 2, no thermals): 26,103 26.9,103 27,103 27.4,103.4 28.9,103.4 28.9,101.6 29.7,100.8 29.7,100.1 29.5,99.9 29.3,99.9 28.6,100.6 28.6,101.6 27.4,101.6 27,102 26,102
N$1  (via drill 0.3)
  Top 0.152: R7.2 42.7,86.5 v43.3,87.1 | 60.9,109.2 J16.GRNN 60.9,108.38 59.59,107.08 59.59,101.5 59.7,101.4 v59.7,99.4
  Bottom 0.152: v43.3,87.1 45,88.8 45,89.32 45.76,90.08 45.76,93.08 45.42,93.41 45.42,96.46 49.23,100.26 58.84,100.26 v59.7,99.4
N$2  (via drill 0.3)
  Top 0.152: R8.2 40.2,88.25 41.95,88.25 42.4,88.7 v43.4,88.7
  Bottom 0.152: v43.4,88.7 44.25,89.55 44.8,89.55 45.45,90.2 45.45,92.95 45.12,93.28 45.12,96.59 49.1,100.57 60.96,100.57 61.5,100.03 61.5,98.53 J16.YLWN
N$3  (via drill 0.3)
  Top 0.152: U8.14 42.52,66.92 v42.9,67.3
  Bottom 0.152: v42.9,67.3 43.98,68.38 54.99,68.38 59.4,63.98 J18.P$6
N$4  (via drill 0.3)
  Top 0.152: U8.13 41.27,66.5 42.92,66.5 43.72,67.3 v43.76,67.3
  Bottom 0.152: v43.76,67.3 43.76,67.73 44.11,68.08 54.87,68.08 59.27,63.67 64.63,63.67 65.3,63 66.06,63 66.66,63.59 66.66,64.15 J18.P$5
N$5  (via drill 0.3)
  Top 0.152: R24.1 33.27,64.33 U8.7 36.58,64.33 37.49,65.23 37.49,65.5 37.88,65.9 v37.88,66.75
  Bottom 0.152: v37.88,66.75 37.6,67.02 37.6,68.27 38.02,68.69 55.12,68.69 59.53,64.28 63.99,64.28 J18.P$4
N$6  (via drill 0.3)
  Top 0.152: R24.2 33.98,64.97 U8.6 36.8,64.97 37.18,65.36 37.18,66.08 v37.26,66.16
  Bottom 0.152: v37.26,66.16 37.3,66.2 37.3,68.4 37.89,68.99 55.25,68.99 59.65,64.59 63.87,64.59 64.79,65.51 64.79,66.39 65.42,67.02 J18.P$3
N$7  (via drill 0.3)
  Top 0.152: R23.1 33.02,67.58 U8.2 35.37,67.8 36.05,67.8 36.18,67.93 36.18,68.6 36.32,68.74 v36.49,68.74 | v62.7,65.17 62.7,64.97 J18.P$8
  Bottom 0.152: v36.49,68.74 36.77,69.02 36.84,69.02 37.12,69.3 55.37,69.3 59.78,64.89 62.4,64.89 62.68,65.17 v62.7,65.17
N$8  (via drill 0.3)
  Top 0.152: R23.2 34.23,68.22 U8.1 36.52,69.6 v36.6,69.6 | v63.56,65.17 63.56,64.54 65.14,62.96 J18.P$7
  Bottom 0.152: v36.6,69.6 55.5,69.6 59.91,65.19 61.91,65.19 62.46,65.75 62.98,65.75 v63.56,65.17
N$9  (via drill 0.3)
  Top 0.152: U8.11 43.38,64.97 v43.5,65.1 | v56.71,65.41 62.12,65.41 62.46,65.75 63.43,65.75 J18.P$2
  Bottom 0.152: v43.5,65.1 46.17,67.77 54.74,67.77 56.71,65.8 v56.71,65.41
N$10  (via drill 0.3)
  Top 0.152: U8.10 43.55,64.33 v44.36,65.14 | v55.89,65.8 56.28,65.8 56.47,65.99 56.95,65.99 57.23,65.72 61.99,65.72 62.33,66.05 63.3,66.05 64.79,67.54 64.79,68.43 65.42,69.06 J18.P$1
  Bottom 0.152: v44.36,65.14 44.36,65.53 46.3,67.47 54.62,67.47 55.89,66.19 v55.89,65.8
N$13
  Top 0.152: U3.58 12.55,61.9 Y1.1
N$14
  Top 0.152: Y1.3 11.47,61.68 11.47,61.35 11.61,61.22 11.93,61.22 12.05,61.1 U3.59
N$15
  Top 0.152: D6.2 R6.2
N$17
  Top 0.152: D5.2 R5.2
N$19
  Top 0.152: U5.9 26.7,23.25 R1.2
N$21
  Top 0.152: D4.2 R4.2
N$25  (via drill 0.3)
  Top 0.152: U7.14 42.62,79.42 v42.9,79.7
  Bottom 0.152: v42.9,79.7 44.78,81.58 64.65,81.58 64.87,81.81 65.05,81.81 J17.P$6
N$26  (via drill 0.3)
  Top 0.152: U7.13 41.27,79 43.02,79 v43.76,79.74
  Bottom 0.152: v43.76,79.74 43.76,80.06 44.98,81.28 63.9,81.28 64.78,81.28 65,81.5 66.06,81.5 67.5,82.94 J17.P$5
N$27  (via drill 0.3)
  Top 0.152: R22.1 33.27,76.83 U7.7 36.68,76.83 37.59,77.73 37.59,78.47 37.41,78.65 37.41,78.97 v37.96,79.53
  Bottom 0.152: v37.96,79.53 37.96,79.88 38.55,80.47 38.55,81.25 39.18,81.89 64.19,81.89 64.7,82.4 64.7,83.5 65.71,84.51 J17.P$4
N$28  (via drill 0.3)
  Top 0.152: R22.2 33.98,77.47 U7.6 35.19,77.52 36.94,77.52 37.28,77.86 37.28,78.34 37.1,78.52 v37.1,79.49
  Bottom 0.152: v37.1,79.49 37.86,80.26 37.9,80.26 38.24,80.6 38.24,81.38 39.05,82.19 64.06,82.19 64.39,82.53 64.39,84.5 65.42,85.52 J17.P$3
N$29  (via drill 0.3)
  Top 0.152: R21.1 33.02,80.08 U7.2 36.9,80.08 v37.66,80.84 | v62.9,82.77 65.23,80.44 J17.P$8
  Bottom 0.152: v37.66,80.84 37.66,81.23 38.93,82.5 62.62,82.5 v62.9,82.77
N$30  (via drill 0.3)
  Top 0.152: R21.2 34.23,80.72 U7.1 36.73,80.72 v36.8,80.8 | v63.76,82.77 65.07,81.46 J17.P$7
  Bottom 0.152: v36.8,80.8 38.8,82.8 62.1,82.8 62.66,83.35 63.18,83.35 v63.76,82.77
N$31  (via drill 0.3)
  Top 0.152: U7.11 43.27,77.47 v43.5,77.7 | v63,80.69 63,81.7 62,82.7 62,83.5 65.04,86.54 J17.P$2
  Bottom 0.152: v43.5,77.7 44.34,78.54 44.34,80.21 45.1,80.97 61.1,80.97 | 61.1,80.97 | 61.1,80.97 62.8,80.97 63,80.77 v63,80.69
N$32  (via drill 0.3)
  Top 0.152: v43.5,76.84 41.07,76.84 U7.10 | v62.14,80.39 62.42,80.67 62.42,80.94 62.7,81.21 62.7,81.57 61.7,82.57 61.7,83.63 64.79,86.72 64.79,86.93 65.42,87.56 J17.P$1
  Bottom 0.152: v43.5,76.84 43.5,76.88 44.08,77.46 44.08,77.85 44.65,78.41 44.65,80.08 45.23,80.67 61.86,80.67 v62.14,80.39
N$33  (via drill 0.3)
  Top 0.152: R9.2 44,75.95 v44.25,75.95 | J17.GRNN 59.6,89.56 v59.6,79.78
  Bottom 0.152: v44.25,75.95 44.62,76.32 44.64,76.32 44.98,76.66 44.98,77.14 44.7,77.42 44.7,77.61 45.26,78.16 45.26,79.83 45.48,80.06 59.32,80.06 v59.6,79.78
N$34  (via drill 0.3)
  Top 0.152: R10.2 40.2,75.75 43.23,75.75 44.38,76.9 v44.4,76.9
  Bottom 0.152: v44.4,76.9 44.4,77.74 44.95,78.29 44.95,79.96 45.35,80.36 59.96,80.36 J17.YLWN
N$35  (via drill 0.3)
  Top 0.152: R11.2 43.15,62.7 v43.3,62.7 | v54.51,66.31 54.85,66.31 J18.GRNN
  Bottom 0.152: v43.3,62.7 43.3,63.37 44.18,64.25 44.73,64.25 45.25,64.77 45.25,65.56 46.55,66.86 54.2,66.86 54.51,66.54 v54.51,66.31
N$36  (via drill 0.3)
  Top 0.152: R12.2 39.85,62.9 v42.4,62.9
  Bottom 0.152: v42.4,62.9 44.06,64.56 44.6,64.56 44.94,64.9 44.94,65.68 46.42,67.16 54.49,67.16 55.31,66.34 55.31,65.56 59.94,60.93 J18.YLWN
N$37
  Top 0.152: D2.2 R2.2
N$38
  Top 0.152: D3.2 R3.2
N$39  (via drill 0.3)
  Top 0.152: U9.14 42.23,54.92 v42.8,55.5
  Bottom 0.152: v42.8,55.5 43.58,56.28 48.59,56.28 59.4,45.48 J19.P$6
N$40  (via drill 0.3)
  Top 0.152: U9.13 42.63,54.27 v43,54.64
  Bottom 0.152: v43,54.64 43,54.88 43.38,55.26 43.38,55.65 43.71,55.98 48.47,55.98 59.27,45.17 64.6,45.17 65.27,44.5 66.06,44.5 67.5,45.94 J19.P$5
N$41  (via drill 0.3)
  Top 0.152: R26.1 33.27,52.33 U9.7 36.58,52.33 37.59,53.33 37.59,54.07 37.54,54.11 37.54,54.74 37.82,55.02 37.82,55.81 v37.86,55.85
  Bottom 0.152: v37.86,55.85 37.8,55.91 37.8,56.18 37.81,56.19 37.81,56.59 48.72,56.59 57.8,47.51 J19.P$4
N$42  (via drill 0.3)
  Top 0.152: R26.2 33.98,52.98 U9.6 35.29,53.12 36.94,53.12 37.28,53.46 37.28,53.94 37.24,53.99 v37.24,55.26
  Bottom 0.152: v37.24,55.26 37.24,56.05 37.51,56.31 37.51,56.74 37.65,56.89 48.85,56.89 57.92,47.81 64.71,47.81 65.34,48.44 67.42,48.44 J19.P$3
N$43  (via drill 0.3)
  Top 0.152: R25.1 35.12,55.55 U9.2 36.33,55.58 v36.6,55.84 | v62.2,48.4 64.1,46.49 64.1,44.6 65.26,43.44 J19.P$8
  Bottom 0.152: v36.6,55.84 37.2,56.44 37.2,56.87 37.53,57.2 48.97,57.2 58.05,48.12 61.92,48.12 v62.2,48.4
N$44  (via drill 0.3)
  Top 0.152: R25.2 34.23,56.23 U9.1 36.12,56.23 v36.6,56.7 | v61.34,48.7 61.68,48.7 61.96,48.98 62.44,48.98 62.78,48.64 62.78,48.24 64.41,46.62 64.41,44.73 64.72,44.42 67.46,44.42 J19.P$7
  Bottom 0.152: v36.6,56.7 37.4,57.5 49.1,57.5 58.18,48.42 61.06,48.42 v61.34,48.7
N$45  (via drill 0.3)
  Top 0.152: U9.11 43.17,52.98 v43.5,53.3 | v57.46,46.16 60.84,49.54 J19.P$2
  Bottom 0.152: v43.5,53.3 43.7,53.5 43.7,55.54 43.83,55.67 48.34,55.67 56.34,47.67 | 56.34,47.67 | v57.46,46.16 57.46,46.55 56.34,47.67
N$46  (via drill 0.3)
  Top 0.152: U9.10 43.74,52.33 v43.91,52.49 | v56.64,46.55 56.88,46.8 57.67,46.8 60.71,49.84 64.64,49.84 65.4,50.6 67.46,50.6 J19.P$1
  Bottom 0.152: v43.91,52.49 43.91,52.88 44.08,53.06 44.08,53.54 44.01,53.62 44.01,55.27 44.1,55.37 48.22,55.37 56.22,47.37 | 56.22,47.37 | 56.22,47.37 56.64,46.94 v56.64,46.55
N$47  (via drill 0.3)
  Top 0.152: R13.2 42.62,50.17 v43.23,50.17 | v54.46,47.86 60.46,53.86 J19.GRNN
  Bottom 0.152: v43.23,50.17 43.23,50.56 44.79,52.12 44.79,53.69 44.61,53.87 44.61,54.76 47.96,54.76 54.46,48.26 v54.46,47.86
N$48  (via drill 0.3)
  Top 0.152: R14.2 38.45,49.75 v39.1,50.4
  Bottom 0.152: v39.1,50.4 42.64,50.4 44.49,52.25 44.49,53.56 44.31,53.74 44.31,55.06 48.09,55.06 56.06,47.09 56.06,46.31 59.94,42.43 J19.YLWN
N$49  (via drill 0.3)
  Top 0.152: U10.14 42.73,41.92 v43.1,42.3
  Bottom 0.152: v43.1,42.3 44.48,43.68 48.4,43.68 | 48.4,43.68 | 48.4,43.68 57.8,34.28 57.8,31.9 62.72,26.98 J20.P$6
N$50  (via drill 0.3)
  Top 0.152: U10.13 42.9,41.27 v43.96,42.34
  Bottom 0.152: v43.96,42.34 43.96,42.73 44.61,43.38 48.27,43.38 57.49,34.15 57.49,31.77 62.6,26.67 64.33,26.67 64.96,26.04 66.11,26.04 66.66,26.59 66.66,27.15 J20.P$5
N$51  (via drill 0.3)
  Top 0.152: R28.1 33.27,39.33 U10.7 36.78,39.33 38.19,40.74 38.19,43.12 v38.78,43.71 v38.79,43.71
  Bottom 0.152: v38.79,43.71 39.07,43.99 48.52,43.99 58.1,34.4 58.1,32.03 61.12,29.01 J20.P$4
N$52  (via drill 0.3)
  Top 0.152: R28.2 33.98,39.98 U10.6 35.29,40.12 37.14,40.12 37.89,40.87 37.89,43.33 37.71,43.51 37.77,43.51 v37.93,43.68
  Bottom 0.152: v37.93,43.68 37.93,44.02 38.2,44.29 48.65,44.29 58.41,34.53 58.41,32.15 61.25,29.31 64.61,29.31 65.3,30 67.48,30 J20.P$3
N$53  (via drill 0.3)
  Top 0.152: R27.1 33.02,42.58 U10.2 36.08,42.58 36.42,42.92 36.74,42.92 36.92,43.09 v37.31,43.09 | v63.6,29.89 63.6,27.07 J20.P$8
  Bottom 0.152: v37.31,43.09 37.31,43.88 38.03,44.59 48.77,44.59 58.71,34.66 58.71,32.28 61.38,29.62 63.4,29.62 63.6,29.82 v63.6,29.89
N$54  (via drill 0.3)
  Top 0.152: R27.2 34.23,43.23 U10.1 36.23,43.23 v36.5,43.5 | v64.46,29.98 64.18,29.7 64.18,29.65 63.91,29.38 63.91,27.19 65.14,25.96 J20.P$7
  Bottom 0.152: v36.5,43.5 37.9,44.9 48.9,44.9 59.02,34.78 59.02,32.41 61.5,29.92 62.8,29.92 63.36,30.48 63.84,30.48 64.39,29.92 64.4,29.92 v64.46,29.98
N$55  (via drill 0.3)
  Top 0.152: U10.11 43.58,39.98 v43.9,40.3 | v60.42,28.02 63.44,31.04 J20.P$2
  Bottom 0.152: v43.9,40.3 44.54,40.94 44.54,42.58 44.53,42.59 44.53,42.87 44.73,43.07 48.14,43.07 57.19,34.02 57.19,31.65 60.22,28.62 60.22,28.23 v60.42,28.02
N$56  (via drill 0.3)
  Top 0.152: U10.10 43.78,39.33 v44.76,40.3 | v61.03,27.42 61.03,28.2 63.57,30.73 64.71,30.73 65.34,30.11 66.11,30.11 66.66,30.65 66.66,31.21 J20.P$1
  Bottom 0.152: v44.76,40.3 44.6,40.46 44.6,40.57 44.84,40.81 44.84,42.75 44.86,42.77 48.02,42.77 56.89,33.9 56.89,31.52 59.84,28.57 59.84,27.78 60.21,27.42 v61.03,27.42
N$57  (via drill 0.3)
  Top 0.152: R15.2 43.16,37.71 v43.16,37.94 | v56,33.1 58.26,35.36 J20.GRNN
  Bottom 0.152: v43.16,37.94 43.16,38.33 44.24,39.41 45.13,39.41 45.65,39.93 45.65,40.67 45.45,40.86 45.45,42.16 47.76,42.16 56.01,33.91 56.01,33.11 v56,33.1
N$58  (via drill 0.3)
  Top 0.152: R16.2 39.85,37.9 v42.3,37.9
  Bottom 0.152: v42.3,37.9 44.12,39.72 45,39.72 45.34,40.06 45.34,40.54 45.15,40.73 45.15,42.46 47.89,42.46 56.58,33.77 56.58,31.39 59.54,28.44 59.54,27.66 60.8,26.39 60.8,24.02 J20.YLWN
N$59  (via drill 0.3)
  Top 0.152: U11.14 43.02,28.93 v43.1,29
  Bottom 0.152: v43.1,29 46.08,29 48,27.08 48,21.1 60.62,8.48 J21.P$6
N$60  (via drill 0.3)
  Top 0.152: U11.13 41.17,28.39 v43.71,28.39
  Bottom 0.152: v43.71,28.39 44.01,28.7 45.95,28.7 47.7,26.95 47.7,20.97 60.5,8.17 64.71,8.17 65.34,7.54 66.11,7.54 66.66,8.09 66.66,8.65 J21.P$5
N$61  (via drill 0.3)
  Top 0.152: R30.1 33.27,26.32 U11.7 36.58,26.32 37.63,27.37 37.63,29.45 v38.18,30
  Bottom 0.152: v38.18,30 38.18,30.41 38.24,30.47 38.24,31 38.43,31.19 44.32,31.19 48.3,27.2 48.3,21.23 59.02,10.51 J21.P$4
N$62  (via drill 0.3)
  Top 0.152: R30.2 33.98,26.98 U11.6 35.29,27.12 36.94,27.12 37.32,27.5 v37.32,29.98
  Bottom 0.152: v37.32,29.98 37.94,30.59 37.94,31.13 38.3,31.49 44.45,31.49 48.61,27.33 48.61,21.35 59.15,10.81 64.71,10.81 65.39,11.5 67.48,11.5 J21.P$3
N$63  (via drill 0.3)
  Top 0.152: R29.1 33.02,29.57 U11.2 36.1,29.57 v37.36,30.84 | v63,11.39 63.7,10.7 63.7,7.8 65.06,6.44 J21.P$8
  Bottom 0.152: v37.36,30.84 37.36,31.23 37.93,31.8 44.57,31.8 48.91,27.45 48.91,21.48 59.28,11.12 62.72,11.12 v63,11.39
N$64  (via drill 0.3)
  Top 0.152: R29.2 34.23,30.23 U11.1 35.92,30.23 v36.5,30.8 | v63.86,11.39 63.8,11.34 63.8,11.03 64,10.82 64,7.93 64.47,7.46 J21.P$7
  Bottom 0.152: v36.5,30.8 37.8,32.1 44.7,32.1 49.22,27.58 49.22,21.61 59.4,11.42 62.2,11.42 62.76,11.98 63.28,11.98 v63.86,11.39
N$65  (via drill 0.3)
  Top 0.152: U11.11 43.48,26.98 v43.6,27.1 | v61.6,7.59 61.6,11.6 62.6,12.6 65.66,12.6 J21.P$2
  Bottom 0.152: v43.6,27.1 44.89,28.39 45.82,28.39 47.39,26.82 47.39,20.85 60.37,7.87 61.3,7.87 61.58,7.59 v61.6,7.59
N$66  (via drill 0.3)
  Top 0.152: U11.10 43.02,26.32 v43.09,26.39 | J21.P$1 65.26,13.56 64.61,12.91 62.47,12.91 61.3,11.73 61.3,8.11 61.02,7.83 61.02,7.56 v60.74,7.29
  Bottom 0.152: v43.09,26.39 43.22,26.52 43.84,26.52 44.18,26.86 44.18,27.25 45.02,28.09 45.7,28.09 47.09,26.7 47.09,20.72 60.24,7.56 60.46,7.56 v60.74,7.29
N$67  (via drill 0.3)
  Top 0.152: v44.57,25.99 44.44,25.99 44.29,25.84 44.29,25.55 43.95,25.21 43.66,25.21 R17.2 | v55.13,11.43 60.56,16.86 J21.GRNN
  Bottom 0.152: v44.57,25.99 44.57,26.38 44.79,26.61 44.79,27 45.27,27.48 45.44,27.48 46.48,26.44 46.48,20.47 55.13,11.82 v55.13,11.43
N$68  (via drill 0.3)
  Top 0.152: v43.71,25.79 42.24,24.33 39.6,24.33 38.78,23.5 R18.2
  Bottom 0.152: v43.71,25.79 43.71,25.95 44.49,26.73 44.49,27.12 45.14,27.78 45.57,27.78 46.78,26.57 46.78,20.59 60.16,7.22 60.16,7.04 60.5,6.7 60.67,6.7 60.9,6.48 J21.YLWN
N$69  (via drill 0.45)
  Top 0.406: S2.P$1 S2.P$4 19.2,105.5 19.2,89.2 v12.8,82.8 | C21.2 J15.P$1
  Bottom 0.406: v12.8,82.8 5.7,75.7 J15.P$1
PDI_DATA
  Top 0.152: J5.1 9.16,87.34 11,85.5 11,67.2 13.8,64.4 13.8,60.7 13.55,60.45 U3.56
RESET/PDI_CLK
  Top 0.152: U3.57 13.05,60.38 13.49,60.83 13.49,63.51 12.4,64.6 10.1,66.9 10.1,85 8.1,87 8.1,96.4 | 8.1,96.4 8.1,97.7 8.5,98.1 12.59,98.1 J5.5 | S1.P$4 2.2,97.5 3.3,96.4 8.1,96.4
RX-A  (via drill 0.3)
  Top 0.152: R20.2 33.48,89.97 U6.6 35.19,90.02 37.14,90.02 38.02,90.9 38.1,90.9 38.1,91.2 v38.04,91.26
  Bottom 0.152: v38.04,91.26 38.26,91.26 38.61,91.61 38.61,92.67 48.34,102.39 63.3,102.39 64.93,104.02 J16.P$3
RX-B  (via drill 0.3)
  Top 0.152: R20.1 33.77,89.33 U6.7 36.92,89.33 v37,89.4
  Bottom 0.152: v37,89.4 38.92,91.32 38.92,92.54 48.47,102.09 63.82,102.09 64.37,102.64 65.36,102.64 J16.P$4
STLCLK  (via drill 0.3)
  Top 0.152: R5.1 10.45,104.3 v8,104.3 | v7.4,95.7 7.4,94.8 7.79,94.41 7.79,86.87 9.79,84.87 9.79,61.91 10.55,61.15 U3.62
  Bottom 0.152: v8,104.3 7.4,103.7 v7.4,95.7
STLERR  (via drill 0.3)
  Top 0.152: v6.82,95.07 7.09,94.79 7.09,94.67 7.49,94.28 7.49,86.75 9.49,84.75 9.49,61.78 10.05,61.22 U3.63 | v7.14,104.26 7.9,105.02 R4.1
  Bottom 0.152: v6.82,95.07 6.82,95.94 7.09,96.22 7.09,104.22 v7.14,104.26
TX-Y  (via drill 0.3)
  Top 0.152: U6.14 42.92,91.92 v43.4,92.4 | v64.61,102.06 65.7,100.98 J16.P$6
  Bottom 0.152: v43.4,92.4 43.9,92.9 43.9,97.09 48.59,101.78 64.42,101.78 64.42,101.87 v64.61,102.06
TX-Z  (via drill 0.3)
  Top 0.152: U6.13 43.1,91.28 v44.26,92.44
  Bottom 0.152: v44.26,92.44 44.1,92.59 44.1,92.67 44.2,92.77 44.2,96.97 48.72,101.48 64.91,101.48 65.34,101.91 67.42,101.91 J16.P$5
VCC  (via drill 0.3)
  Top 0.254: U4.11 27.75,104.85 v27.8,104.9
  Top 1.27: J8.P$1 36.5,106.7 v33.4,103.6 | v33.4,103.6 33.4,103.2 | v33.4,103.6 33.4,101.8 30.8,99.2 29.1,99.2 29.1,98.7 C12.1
  Bottom 0.254: v27.8,104.9 32.1,104.9 v33.4,103.6
  pour Top (rank 3, no thermals): 27.5,101.5 28.5,101.5 28.5,100.5 29.3,99.7 29.8,99.7 29.8,99 29.2,99 28.6,98.4 28.3,98.4 28.3,99.2 27.5,100
VSW  (via drill 0.3)
  Top 0.254: U4.12 27.25,104.56 27.17,104.64 27.17,105.53 C15.1
  other vias: 26.9,97.8 26.2,98.9 27.7,98.9 27.7,96.9 26.1,96.9
  pour Top (no thermals): 27.4,104.5 27.4,103.6 26.9,103.1 25.9,103.1 25.9,101.9 26.9,101.9 27.4,101.4 27.4,100.2 27.4,100 28.2,99.2 28.2,96.5 25.7,96.5 25.7,99.3 25.2,99.8 22.9,99.8 22.9,104.6 24.5,106.2 27.3,106.2 27.3,104.7 27.3,104.6
  pour Bottom: 25.4,96.3 23.2,96.3 23.2,99.6 32.5,99.6 32.5,96.3

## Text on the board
tPlace: err | clk | pwr | < pwr rpi | pwr brd > | VCC | GND | reset | ATKP0 | ATKP1 | < pwr to rpi | ATKP2 | atkrouter v0.21 / https://gitlab.cba.mit.edu/jakeread/automatakit | ATKP3 | rx atk | ATKP4 | tx atk | usbdm | usbdp | gnd > | < pwr from rpi | cut for no usb power from host | ATKP5 | rx bridge | tx bridge
bPlace: big open spaces / are like endless durations / until you find it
